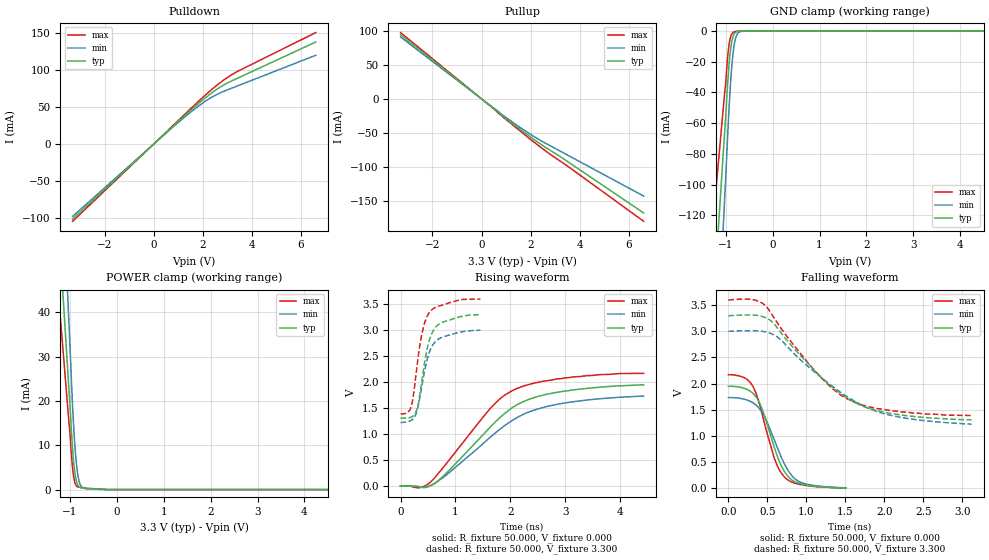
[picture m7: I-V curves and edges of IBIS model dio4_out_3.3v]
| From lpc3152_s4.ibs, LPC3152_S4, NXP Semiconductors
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[Model]   dio4_out_3.3v
Model_type Output
Vref=0.000E+00
Rref=1.000E+06
Cref=2.500E-11
Vmeas=1.650E+00
C_comp   1.080E-12   1.060E-12   1.100E-12
[Voltage Range]   3.300E+00   3.000E+00   3.600E+00
[POWER Clamp Reference]   3.300E+00   3.000E+00   3.600E+00
[GND Clamp Reference]   0.000E+00   0.000E+00   0.000E+00
[Pullup Reference]   3.300E+00   3.000E+00   3.600E+00
[Pulldown Reference]   0.000E+00   0.000E+00   0.000E+00
[Temperature Range]   25   85   -40
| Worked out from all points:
|   slope of the pulldown table from 0 to 0.495 V, typ, clamps not added: 32.6 ohm
|   slope of the pullup table from 0 to 0.495 V, typ, clamps not added: 35.1 ohm
|   GND clamp passes 1 mA (typ) near -0.79 V on its own axis
|   POWER clamp passes 1 mA (typ) near -0.83 V on its own axis
|   rising waveform, R_fixture 50.000, V_fixture 0.000: 20-80 % time 1.15ns typ, 1.26ns min, 1.04ns max; typ from 0 V to 1.95 V
|   falling waveform, R_fixture 50.000, V_fixture 0.000: 20-80 % time 272ps typ, 305ps min, 253ps max; typ from 1.95 V to 0 V
|   rising waveform, R_fixture 50.000, V_fixture 3.300: 20-80 % time 211ps typ, 221ps min, 197ps max; typ from 1.3 V to 3.3 V
|   falling waveform, R_fixture 50.000, V_fixture 3.300: 20-80 % time 830ps typ, 924ps min, 767ps max; typ from 3.3 V to 1.3 V
[GND Clamp]
-3.3V     -1.134A    -1.536A    -813.9mA
-1.02V    -64.74mA   -108.1mA   -39.73mA
-1V       -56.46mA   -96.14mA   -34.47mA
-960mV    -35.45mA   -69.89mA   -17.76mA
-920mV    -19.08mA   -46.14mA   -7.381mA
-880mV    -8.715mA   -27.11mA   -2.671mA
-860mV    -5.565mA   -19.78mA   -1.61mA
-820mV    -2.098mA   -9.475mA   -660.7uA
-780mV    -810.7uA   -3.971mA   -358uA
-740mV    -390.5uA   -1.546mA   -274.6uA
-600mV    -206.8uA   -209.1uA   -224.9uA
6.6V      0A         0A         0A
[Power Clamp]
-3.3V     407.9mA    577.3mA    309.6mA
-1.02V    22.73mA    37.76mA    15.33mA
-1V       19.74mA    33.38mA    13.18mA
-960mV    12.15mA    23.16mA    7.084mA
-920mV    6.315mA    14.53mA    2.952mA
-880mV    2.898mA    8.225mA    1.181mA
-840mV    1.3mA      4.096mA    641.8uA
-820mV    878.4uA    2.747mA    562.7uA
-780mV    487.3uA    1.183mA    498.5uA
-720mV    331.3uA    429.1uA    415uA
-380mV    112.1uA    57.06uA    148uA
6.6V      0A         0A         0A
[Pullup]
-3.3V     94.69mA    91.37mA    97.9mA
800mV     -23.6mA    -22.36mA   -24.43mA
1.86V     -52.71mA   -49.26mA   -55.95mA
2.6V      -71.51mA   -65.42mA   -76.57mA
3.16V     -84.09mA   -76.28mA   -90.81mA
6.6V      -168.4mA   -143.5mA   -180.7mA
[Pulldown]
-3.3V     -101.3mA   -97.68mA   -104.3mA
1V        30.74mA    29.33mA    31.89mA
1.48V     45.06mA    42.56mA    47.12mA
2.16V     64.02mA    59.23mA    67.86mA
2.82V     79.28mA    70.94mA    85.83mA
3.3V      87.3mA     77.18mA    96.28mA
6.6V      138mA      120.1mA    150.7mA
[Rising Waveform]
R_fixture = 50.000
V_fixture = 0.000
V_fixture_min = 0.000
V_fixture_max = 0.000
|  time   V(typ)   V(min)   V(max)
0s        0V         0V         0V
350ps     -20.87mV   -15.95mV   -34.81mV
485ps     -23.62mV   -13.5mV    23.92mV
630ps     51.17mV    55.29mV    164mV
1.62ns    1.119V     926mV      1.477V
1.87ns    1.373V     1.142V     1.729V
2.1ns     1.55V      1.303V     1.869V
2.42ns    1.698V     1.456V     1.978V
2.91ns    1.814V     1.584V     2.065V
4.425ns   1.947V     1.731V     2.168V
[Falling Waveform]
R_fixture = 50.000
V_fixture = 0.000
V_fixture_min = 0.000
V_fixture_max = 0.000
|  time   V(typ)   V(min)   V(max)
0s        1.947V     1.731V     2.168V
215ps     1.902V     1.694V     2.102V
315ps     1.812V     1.631V     1.942V
360ps     1.732V     1.581V     1.789V
440ps     1.48V      1.428V     1.37V
585ps     791.9mV    933.3mV    582.9mV
730ps     287.5mV    426.7mV    189.2mV
830ps     135.7mV    207mV      100.9mV
945ps     70.43mV    95.63mV    60.59mV
1.51ns    0V         0V         0V
[Rising Waveform]
R_fixture = 50.000
V_fixture = 3.300
V_fixture_min = 3.000
V_fixture_max = 3.600
|  time   V(typ)   V(min)   V(max)
0s        1.305V     1.223V     1.388V
180ps     1.32V      1.254V     1.489V
225ps     1.344V     1.288V     1.679V
285ps     1.438V     1.397V     2.177V
375ps     1.919V     1.839V     2.859V
440ps     2.387V     2.224V     3.149V
520ps     2.793V     2.562V     3.336V
625ps     3.041V     2.77V      3.435V
735ps     3.141V     2.855V     3.476V
1.455ns   3.3V       3V         3.6V
[Falling Waveform]
R_fixture = 50.000
V_fixture = 3.300
V_fixture_min = 3.000
V_fixture_max = 3.600
|  time   V(typ)   V(min)   V(max)
0s        3.3V       3V         3.6V
285ps     3.314V     3.013V     3.615V
460ps     3.272V     2.994V     3.512V
555ps     3.189V     2.953V     3.331V
680ps     2.962V     2.83V      3.048V
1.115ns   2.232V     2.209V     2.233V
1.35ns    1.907V     1.929V     1.883V
1.555ns   1.692V     1.718V     1.684V
2.095ns   1.423V     1.386V     1.478V
3.12ns    1.305V     1.223V     1.388V
[Ramp]
dV/dt_r   1.1691E+00/1.1419E-09   1.0381E+00/1.2573E-09   1.3012E+00/1.0409E-09
dV/dt_f   1.1968E+00/8.2924E-10   1.0662E+00/9.2441E-10   1.3269E+00/7.6510E-10
R_load = 50
